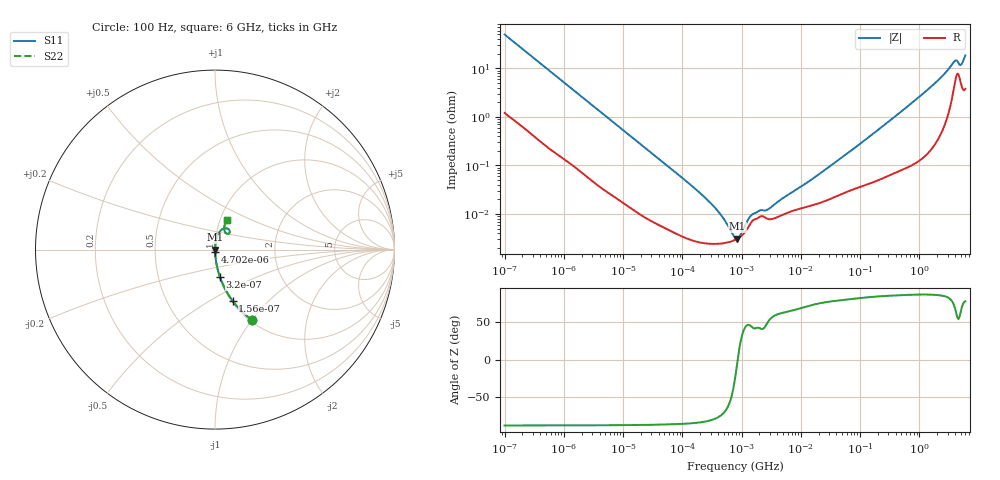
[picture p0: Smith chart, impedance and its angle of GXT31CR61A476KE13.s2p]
!Murata Part Number: GXT31CR61A476KE13
!These Parameters are Measured in Series Mode Connection
!Data Generated on Jan 08, 2026
!  o--ll--o
!Port1  Port2
!  o------o
!Operation Temp=25[degC], DC Bias Voltage=0[V]
!Freq. Start=100[Hz] Stop=6[GHz] 401[Steps]
# Hz S RI R 50
!Freq.(Hz) S11(Real) S11(Imag) S21(Real) S21(Imag) S12(Real) S12(Imag) S22(Real) S22(Imag)
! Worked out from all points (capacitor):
!   401 points, 100 Hz to 6 GHz, reference 50 ohm
!   read as one part in series: C = 31.8 uF near 109 Hz
!   lowest |Z| = 3.11 mohm at 847.2 kHz (marker M1)
!   series resonance near 860.5 kHz, so ESL is about 1.1 nH
!   S11 on the Smith chart (normalised r, x): 100 Hz: 1.02, -1.00; 156 Hz: 1.02, -0.64; 320 Hz: 1.01, -0.32; 4.702 kHz: 1.00, -0.02; 6 GHz: 1.08, +0.36
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100  0.2042 -0.3912  0.7958 0.3912  0.7958 0.3912  0.2042 -0.3912
156  0.0988 -0.2863  0.9012 0.2863  0.9012 0.2863  0.0988 -0.2863
320  0.028 -0.1532  0.972 0.1532  0.972 0.1532  0.028 -0.1532
717  0.00686 -0.0709  0.9931 0.0709  0.9931 0.0709  0.00686 -0.0709
2008  0.00139 -0.0259  0.9986 0.0259  0.9986 0.0259  0.00139 -0.0259
4702  0.000444 -0.0112  0.9996 0.0112  0.9996 0.0112  0.000444 -0.0112
40335  6.11e-05 -0.00136  0.9999 0.00136  0.9999 0.00136  6.11e-05 -0.00136
184852  2.65e-05 -0.000292  1 0.000292  1 0.000292  2.65e-05 -0.000292
432798  2.46e-05 -9.85e-05  1 9.85e-05  1 9.85e-05  2.46e-05 -9.85e-05
774597  2.93e-05 -1.42e-05  1 1.42e-05  1 1.42e-05  2.93e-05 -1.42e-05
847162  3.1e-05 -2.1e-06  1 2.1e-06  1 2.1e-06  3.1e-05 -2.1e-06
1516199  7.19e-05 6.73e-05  0.9999 -6.73e-05  0.9999 -6.73e-05  7.19e-05 6.73e-05
2074311  8.93e-05 7.96e-05  0.9999 -7.96e-05  0.9999 -7.96e-05  8.93e-05 7.96e-05
2713602  8.02e-05 9.2e-05  0.9999 -9.2e-05  0.9999 -9.2e-05  8.02e-05 9.2e-05
1.555665e7  0.000151 0.000503  0.9998 -0.000503  0.9998 -0.000503  0.000151 0.000503
3.124326e8  0.000691 0.00821  0.9993 -0.00821  0.9993 -0.00821  0.000691 0.00821
1.637704e9  0.00411 0.0433  0.9959 -0.0433  0.9959 -0.0433  0.00411 0.0433
2.931063e9  0.0166 0.0854  0.9834 -0.0854  0.9834 -0.0854  0.0166 0.0854
3.8344e9  0.0517 0.118  0.9483 -0.118  0.9483 -0.118  0.0517 0.118
4.193612e9  0.0771 0.1129  0.9229 -0.1129  0.9229 -0.1129  0.0771 0.1129
5.016141e9  0.057 0.0947  0.943 -0.0947  0.943 -0.0947  0.057 0.0947
6e9  0.0648 0.1631  0.9352 -0.1631  0.9352 -0.1631  0.0648 0.1631
